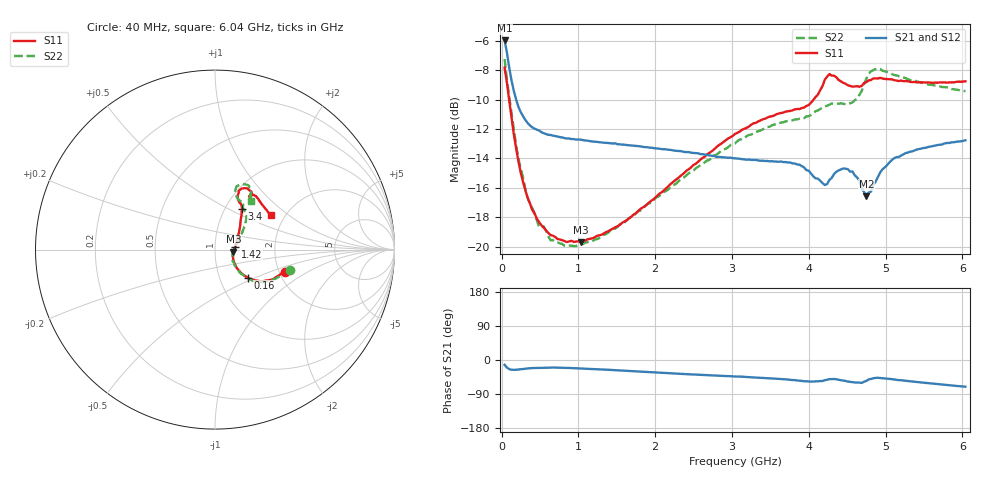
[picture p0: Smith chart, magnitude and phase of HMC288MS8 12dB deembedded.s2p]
!Hittite Microwave Corporation
!12 Elizabeth Drive
!Chelmsford, MA 01824
!Tel: 978-250-3343
!Fax: 978-250-3373
!Device: HMC288MS8, 0.7-3.7 GHz GaAs IC 3-bit Digital Attenuator in 8-lead Grounded Base surface Mount Plastic Package
!Misc:  12dB state, room
# GHZ S DB R 50.0
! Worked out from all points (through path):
!   201 points, 40 MHz to 6.04 GHz, reference 50 ohm
!   highest |S21| = -5.96 dB at 40 MHz (marker M1); lowest = -16.6 dB at 4.75 GHz (marker M2)
!   group delay of S21, straight-line fit = 22.5 ps
!   lowest |S11| = -19.7 dB at 1.03 GHz (marker M3), VSWR 1.23, Z = 61.4 - j1.5 ohm
!   |S11| at or under -10 dB: 98.64 MHz to 4.061 GHz (3.963 GHz wide, 191 % of centre)
!   |S22| runs from -20.0 to -7.2 dB; largest |S21 - S12| = 0.0047
!   S11 on the Smith chart (normalised r, x): 40 MHz: 2.14, -0.63; 160 MHz: 1.36, -0.45; 1.42 GHz: 1.25, +0.04; 3.4 GHz: 1.20, +0.58; 6.04 GHz: 1.70, +0.75
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0.04  -7.82 -17.6  -5.96 -12.8  -5.89 -12.6  -7.23 -15.3
0.1  -10.05 -34.4  -7.80 -24.0  -7.79 -23.8  -9.81 -34.1
0.16  -12.35 -40.6  -9.40 -26.0  -9.39 -26.0  -11.97 -40.4
0.31  -16.16 -39.9  -11.37 -23.1  -11.41 -22.9  -16.08 -39.9
0.49  -18.34 -30.7  -12.10 -21.0  -12.09 -20.6  -18.69 -33.5
0.64  -19.23 -23.9  -12.40 -20.2  -12.40 -20.2  -19.58 -24.0
1.03  -19.70 -6.7  -12.71 -22.2  -12.72 -22.2  -19.81 -6.1
1.06  -19.63 -5.5  -12.75 -22.6  -12.75 -22.5  -19.84 -5.0
1.42  -18.86 8.7  -12.96 -26.1  -12.95 -26.5  -18.91 7.7
2.05  -16.43 31.2  -13.33 -33.2  -13.30 -33.5  -16.57 24.3
3.04  -12.32 52.4  -13.99 -43.5  -13.96 -43.6  -12.97 41.3
3.4  -11.34 56.5  -14.15 -47.1  -14.13 -47.2  -12.03 45.6
3.88  -10.64 61.7  -14.42 -54.7  -14.41 -54.5  -11.29 52.2
4.06  -10.01 66.4  -15.22 -57.0  -15.21 -57.2  -10.92 56.9
4.18  -9.06 68.0  -15.68 -55.6  -15.66 -55.8  -10.56 58.1
4.27  -8.25 61.9  -15.45 -50.3  -15.44 -50.3  -10.34 58.6
4.48  -8.91 55.8  -14.70 -55.3  -14.66 -55.5  -10.31 61.8
4.63  -9.07 56.6  -15.29 -59.5  -15.27 -59.9  -9.94 67.8
4.75  -8.79 57.4  -16.59 -55.3  -16.59 -55.7  -8.57 71.2
4.9  -8.55 53.4  -15.28 -46.9  -15.22 -47.2  -7.89 62.9
5.05  -8.60 50.0  -14.28 -49.8  -14.26 -50.0  -8.13 59.4
6.04  -8.74 31.4  -12.76 -70.6  -12.77 -70.8  -9.41 53.8
